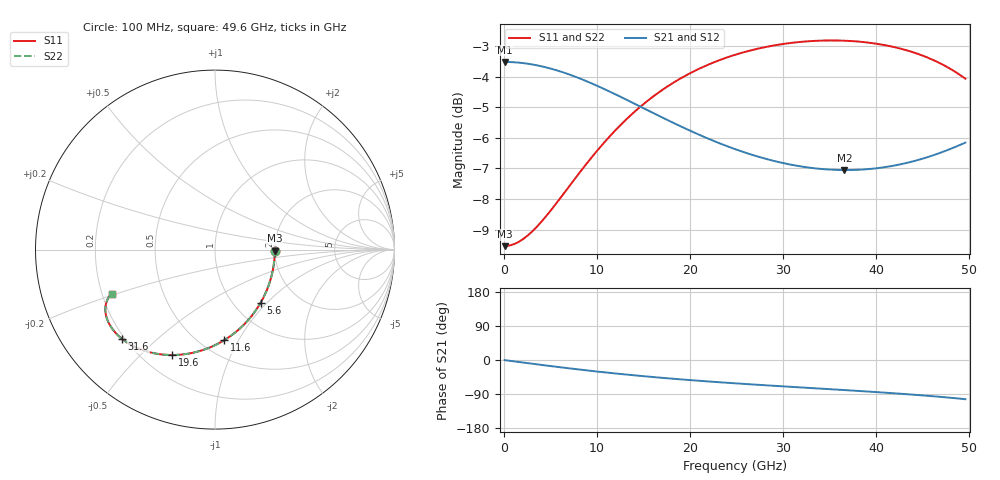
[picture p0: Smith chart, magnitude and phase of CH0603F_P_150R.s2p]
# GHz S RI R 150
! S-Parameters data
! Freq  reS11  imS11  reS21  imS21  reS12  imS12  reS22  imS22
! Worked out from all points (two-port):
!   100 points, 100 MHz to 49.6 GHz, reference 150 ohm
!   highest |S21| = -3.52 dB at 100 MHz (marker M1); lowest = -7.1 dB at 36.6 GHz (marker M2)
!   |S21| within 3 dB of the highest: start of sweep to 26.32 GHz; 46.62 GHz to end of sweep
!   lowest |S11| = -9.5 dB at 100 MHz (marker M3), VSWR 2.00, Z = 300 - j3.83 ohm
!   |S11| at or under -10 dB: nowhere
!   |S22| runs from -9.5 to -2.8 dB; largest |S21 - S12| = 0
!   S11 on the Smith chart (normalised r, x): 100 MHz: 2.00, -0.03; 5.6 GHz: 1.31, -0.92; 11.6 GHz: 0.64, -0.87; 19.6 GHz: 0.32, -0.63; 31.6 GHz: 0.19, -0.39; 49.6 GHz: 0.24, -0.19
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0.1  0.3333 -0.00567  0.6666 -0.00375  0.6666 -0.00375  0.3333 -0.00567
2.6  0.3153 -0.1453  0.6551 -0.0961  0.6551 -0.0961  0.3153 -0.1453
4.1  0.2894 -0.2243  0.6386 -0.1483  0.6386 -0.1483  0.2894 -0.2243
5.6  0.2538 -0.297  0.616 -0.1964  0.616 -0.1964  0.2538 -0.297
7.1  0.2101 -0.3622  0.5886 -0.2396  0.5886 -0.2396  0.2101 -0.3622
8.6  0.1603 -0.4188  0.5575 -0.2773  0.5575 -0.2773  0.1603 -0.4188
10.1  0.1064 -0.4665  0.5242 -0.3095  0.5242 -0.3095  0.1064 -0.4665
11.6  0.0501 -0.5054  0.4898 -0.3364  0.4898 -0.3364  0.0501 -0.5054
14.1  -0.0449 -0.5516  0.4324 -0.3703  0.4324 -0.3703  -0.0449 -0.5516
16.6  -0.1369 -0.5776  0.3776 -0.393  0.3776 -0.393  -0.1369 -0.5776
19.6  -0.2383 -0.5873  0.3176 -0.4095  0.3176 -0.4095  -0.2383 -0.5873
22.6  -0.3275 -0.5797  0.2646 -0.4184  0.2646 -0.4184  -0.3275 -0.5797
25.1  -0.3918 -0.5637  0.2255 -0.4224  0.2255 -0.4224  -0.3918 -0.5637
28.1  -0.4572 -0.5365  0.1836 -0.4254  0.1836 -0.4254  -0.4572 -0.5365
31.6  -0.5183 -0.497  0.1399 -0.4286  0.1399 -0.4286  -0.5183 -0.497
33.1  -0.5397 -0.4783  0.1222 -0.4304  0.1222 -0.4304  -0.5397 -0.4783
36.6  -0.5788 -0.4316  0.082 -0.4362  0.082 -0.4362  -0.5788 -0.4316
39.1  -0.5977 -0.3962  0.0527 -0.4423  0.0527 -0.4423  -0.5977 -0.3962
41.6  -0.6085 -0.3597  0.0214 -0.4499  0.0214 -0.4499  -0.6085 -0.3597
45.6  -0.6068 -0.3002  -0.0372 -0.4648  -0.0372 -0.4648  -0.6068 -0.3002
47.6  -0.5956 -0.2713  -0.0728 -0.4725  -0.0728 -0.4725  -0.5956 -0.2713
49.6  -0.5761 -0.2446  -0.1144 -0.4787  -0.1144 -0.4787  -0.5761 -0.2446
